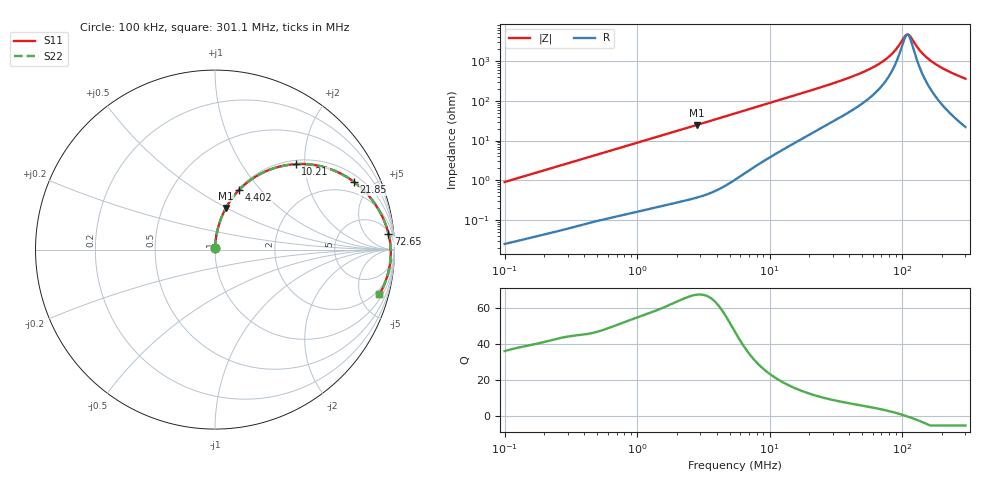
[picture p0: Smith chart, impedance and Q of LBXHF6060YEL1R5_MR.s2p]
! LBXHF6060YEL1R5_MR  S-PARAMETER MODEL  ( General Type )
! Model Generated by TAIYO YUDEN Corporation (http://www.ty-top.com)
! Version 1.0
! TAIYO YUDEN Control No. 200915NI43SB-FBB
! Copyright(c) 2020 TAIYO YUDEN CO.,LTD. All Rights Reserved.
! Product Description (link to TY-COMPAS)
! https://ds.yuden.co.jp/TYCOMPAS/or/detail?pn=LBXHF6060YEL1R5NMR&u=M
! Products Name : Inductors
! Characteristics :
!  Inductance : 1.5 uH , SRF(min) : 77 MHz , DC Resistance(max) : 0.019 Ohm
!  Rated Current : Saturation :10000 mA , Temp Rise : 3400 mA
!  Case Size : 6.0 x 6.0 / 0.236 x 0.236 [mm/inch] , Thickness : 4.5 / 0.177 [mm/inch]
!  (Conditions: Temperature = 25 degC , DC Bias Current/Voltage = 0A / 0V)
! External Node Assignments :
!  1  o---GGG---o  2
! GND o---------o GND
! Frequency Range : 0.1MHz  -  301.082333MHz  [ 402 STEP ]
# MHz S RI R 50
! Freq[MHz].  S11 Real  S11 Imag  S21 Real  S21 Imag  S12 Real  S12 Imag  S22 Real  S22 Imag
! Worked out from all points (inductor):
!   401 points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, 100 kHz to 301.1 MHz, reference 50 ohm
!   read as one part in series: L = 1.44 uH near 104.1 kHz
!   highest Q = 67.3 at 2.834 MHz (marker M1), where L = 1.39 uH
!   self-resonance near 109.7 MHz
!   S11 on the Smith chart (normalised r, x): 100 kHz: 1.00, +0.02; 4.402 MHz: 1.01, +0.77; 10.21 MHz: 1.08, +1.80; 21.85 MHz: 1.33, +3.90; 72.65 MHz: 6, +20; 301.1 MHz: 1.44, -7.24
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0.1  0.000333 0.00906  0.9997 -0.00906  0.9997 -0.00906  0.000333 0.00906
0.382543  0.00192 0.034  0.9981 -0.034  0.9981 -0.034  0.00192 0.034
1.463388  0.0183 0.1258  0.9817 -0.1258  0.9817 -0.1258  0.0183 0.1258
2.833682  0.061 0.232  0.939 -0.232  0.939 -0.232  0.061 0.232
4.402291  0.1342 0.3324  0.8658 -0.3324  0.8658 -0.3324  0.1342 0.3324
5.487097  0.1942 0.385  0.8058 -0.385  0.8058 -0.385  0.1942 0.385
10.208  0.4504 0.4763  0.5496 -0.4763  0.5496 -0.4763  0.4504 0.4763
14.34779  0.611 0.4586  0.389 -0.4586  0.389 -0.4586  0.611 0.4586
20.99048  0.7608 0.3873  0.2392 -0.3873  0.2392 -0.3873  0.7608 0.3873
21.84821  0.7737 0.3779  0.2263 -0.3779  0.2263 -0.3779  0.7737 0.3779
45.83468  0.9272 0.1938  0.0728 -0.1938  0.0728 -0.1938  0.9272 0.1938
59.46364  0.9529 0.1338  0.0471 -0.1338  0.0471 -0.1338  0.9529 0.1338
72.64716  0.9663 0.0894  0.0337 -0.0894  0.0337 -0.0894  0.9663 0.0894
80.29753  0.9711 0.0676  0.0289 -0.0676  0.0289 -0.0676  0.9711 0.0676
90.54875  0.9754 0.0416  0.0246 -0.0416  0.0246 -0.0416  0.9754 0.0416
104.174  0.9785 0.0113  0.0215 -0.0113  0.0215 -0.0113  0.9785 0.0113
110.6241  0.9792 -0.00184  0.0208 0.00184  0.0208 0.00184  0.9792 -0.00184
117.4735  0.9795 -0.015  0.0205 0.015  0.0205 0.015  0.9795 -0.015
140.6728  0.9778 -0.0552  0.0222 0.0552  0.0222 0.0552  0.9778 -0.0552
165.114  0.9731 -0.0923  0.0269 0.0923  0.0269 0.0923  0.9731 -0.0923
214.2107  0.9573 -0.1562  0.0427 0.1562  0.0427 0.1562  0.9573 -0.1562
301.0823  0.9165 -0.2479  0.0835 0.2479  0.0835 0.2479  0.9165 -0.2479
